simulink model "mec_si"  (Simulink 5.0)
settings: Solver=ode45  StartTime=0.0  StopTime=10.0  RelTol=1e-3
libraries: mrlib x1

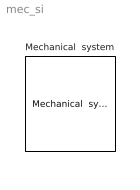
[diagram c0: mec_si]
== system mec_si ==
  Mechanical  system : mrlib/Mechanical  system  H=0.3  Bm=1e-5
